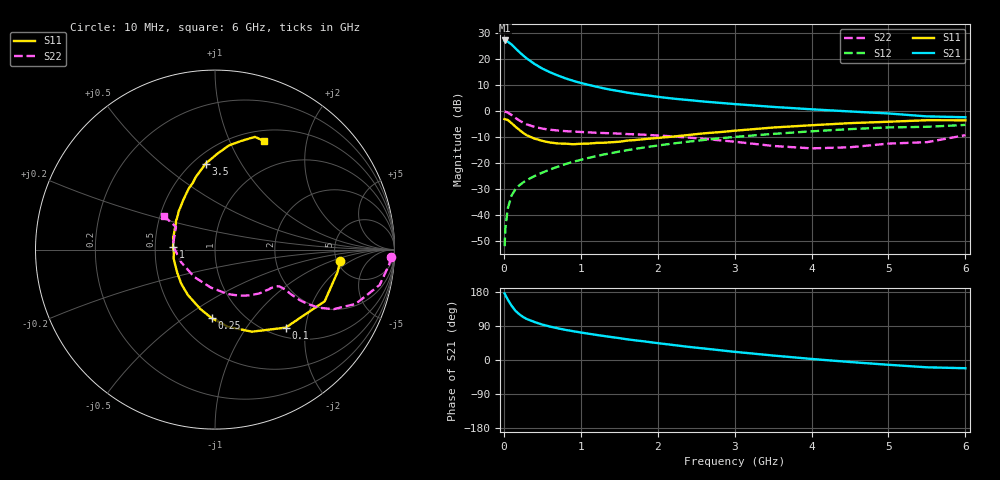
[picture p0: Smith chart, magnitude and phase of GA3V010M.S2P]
! Infineon Technologies  Discrete & RF Semiconductors
! BF775
! Si NPN RF Bipolar Junction Transistor in SOT23
! VCE = 3 V  IC = 10 mA
! Common Emitter S-Parameters:  May  1996
# GHz  S  MA  R  50
!  f  S11  S21  S12  S22
! GHz  MAG  ANG  MAG  ANG  MAG  ANG  MAG  ANG
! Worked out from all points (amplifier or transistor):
!   36 points, 10 MHz to 6 GHz, reference 50 ohm
!   highest |S21| = 27.2 dB at 10 MHz (marker M1)
!   |S21| within 3 dB of that: start of sweep to 149.6 MHz
!   unconditionally stable (mu >= 1): 554.8 MHz to 3.319 GHz
!   at 250 MHz: K = 0.69, MSG = 24.5 dB, |S12| = -27.5 dB
!   at 1.4 GHz: K = 1.12, MAG = 10.1 dB, |S12| = -16.2 dB
!   at 6 GHz: K = 0.96, MSG = 1.5 dB, |S12| = -5.3 dB
!   S11 on the Smith chart (normalised r, x): 10 MHz: 5.32, -1.38; 100 MHz: 1.18, -1.56; 250 MHz: 0.72, -0.64; 1 GHz: 0.62, +0.02; 3.5 GHz: 0.57, +0.72; 6 GHz: 0.63, +1.36
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0.01  0.7008 -5.4  22.91 175.7  0.0025 89.2  0.9826 -2.4
0.02  0.6938 -10.5  22.79 171.4  0.0055 82.5  0.9734 -5.0
0.05  0.6756 -25.2  21.79 160.0  0.0131 78.7  0.9386 -12.1
0.1  0.5866 -47.8  19.17 143.4  0.0235 70.6  0.8404 -21.1
0.15  0.5015 -65.8  16.2 130.0  0.0311 64.1  0.7391 -26.7
0.2  0.4358 -80.4  13.78 120.9  0.037 62.4  0.6612 -29.3
0.25  0.3819 -92.9  11.81 113.5  0.0422 61.3  0.5985 -30.4
0.3  0.3406 -103.9  10.25 108.0  0.047 61.1  0.5531 -30.8
0.4  0.2942 -121.1  8.069 100.2  0.0562 62.2  0.4955 -30.5
0.5  0.267 -135.0  6.58 93.5  0.0652 63.0  0.4595 -29.9
0.6  0.2479 -147.4  5.593 88.3  0.0749 63.9  0.4373 -29.6
0.7  0.238 -158.4  4.858 83.7  0.0848 64.4  0.4228 -29.7
0.8  0.2357 -168.0  4.277 79.6  0.0951 64.2  0.4106 -29.9
1  0.2345 176.5  3.481 72.6  0.115 63.9  0.3958 -31.3
1.1  0.236 169.6  3.202 69.4  0.1253 63.5  0.3892 -32.6
1.3  0.2455 158.4  2.738 63.3  0.1458 62.5  0.3774 -34.8
1.6  0.2696 143.7  2.272 54.7  0.1761 60.1  0.3612 -39.5
2.2  0.3223 124.1  1.738 39.6  0.2375 54.3  0.325 -51.3
3.5  0.482 96.2  1.203 11.8  0.3635 38.3  0.2129 -96.3
4.5  0.5855 82.4  0.983 -5.3  0.4491 25.1  0.2009 -159.3
5.5  0.6662 70.5  0.79 -19.3  0.4977 10.4  0.2516 149.8
6  0.6641 65.5  0.761 -21.7  0.5416 6.3  0.3435 146.6
